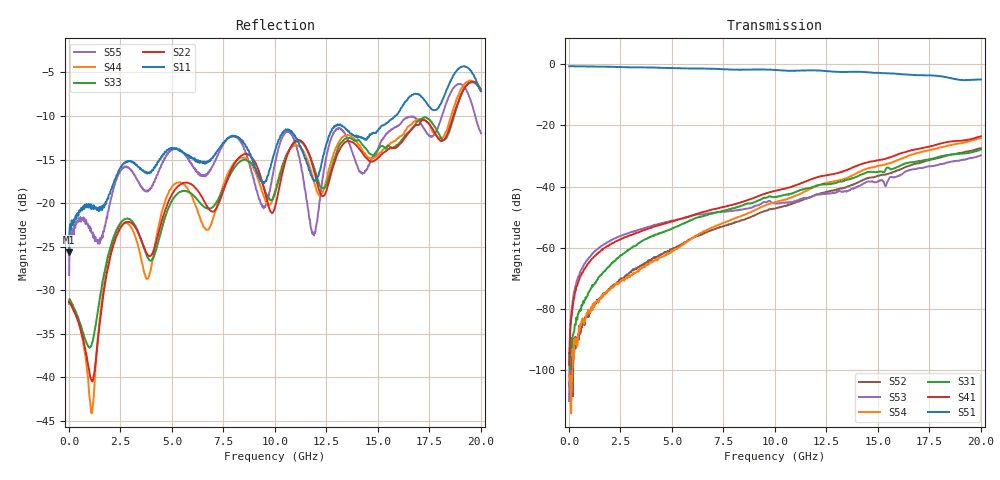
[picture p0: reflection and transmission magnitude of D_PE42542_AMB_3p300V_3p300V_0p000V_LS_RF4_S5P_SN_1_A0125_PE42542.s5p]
! Device ID: PE42542
! Device ID: PE42542
! File Path: z:\PE42542\PE42543_20140723_inv\AMB\3p300\LS_RF4\PE42542_AMB_3p300V_3p300V_0p000V_LS_RF4_S5P_SN_1_A0125_PE42542.s5p
! Serial: 1
! Lot: A0125_PE42542
! Temp: AMB
! VDD: 3.300
! VSS: 0.000
! Control_Hi: 3.300
! Control_Lo: 0.000
! Logic State: LS_RF4
! Port 1: RFC
! Port 2: RF1
! Port 3: RF2
! Port 5: RF3
! Port 6: RF4
! ThroughPath:1-6
! IDD: -0.000142745724
! ISS: 7.65104435e-010
#  Hz  S  RI  R  50
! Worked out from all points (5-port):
!   801 points, 10 MHz to 20 GHz, reference 50 ohm
!   strongest paths, dB at 10 MHz, 5.008 GHz, 10.01 GHz, 15 GHz, 20 GHz:
!     S51: -0.7, -1.4, -1.9, -2.9, -5.0
!     S41: -98.2, -51.3, -41.4, -31.4, -23.6
!     S31: -94.3, -53.7, -43.4, -35.2, -27.9
!     S54: -101.2, -61.2, -45.0, -33.3, -24.2
!     S53: -110.0, -51.2, -45.5, -38.3, -29.8
!     S52: -104.0, -60.4, -47.2, -36.5, -27.4
!   lowest |S11| = -25.7 dB at 10 MHz (marker M1), VSWR 1.11, Z = 55 - j2.22 ohm
!   |S11| at or under -10 dB: start of sweep to 15.84 GHz
